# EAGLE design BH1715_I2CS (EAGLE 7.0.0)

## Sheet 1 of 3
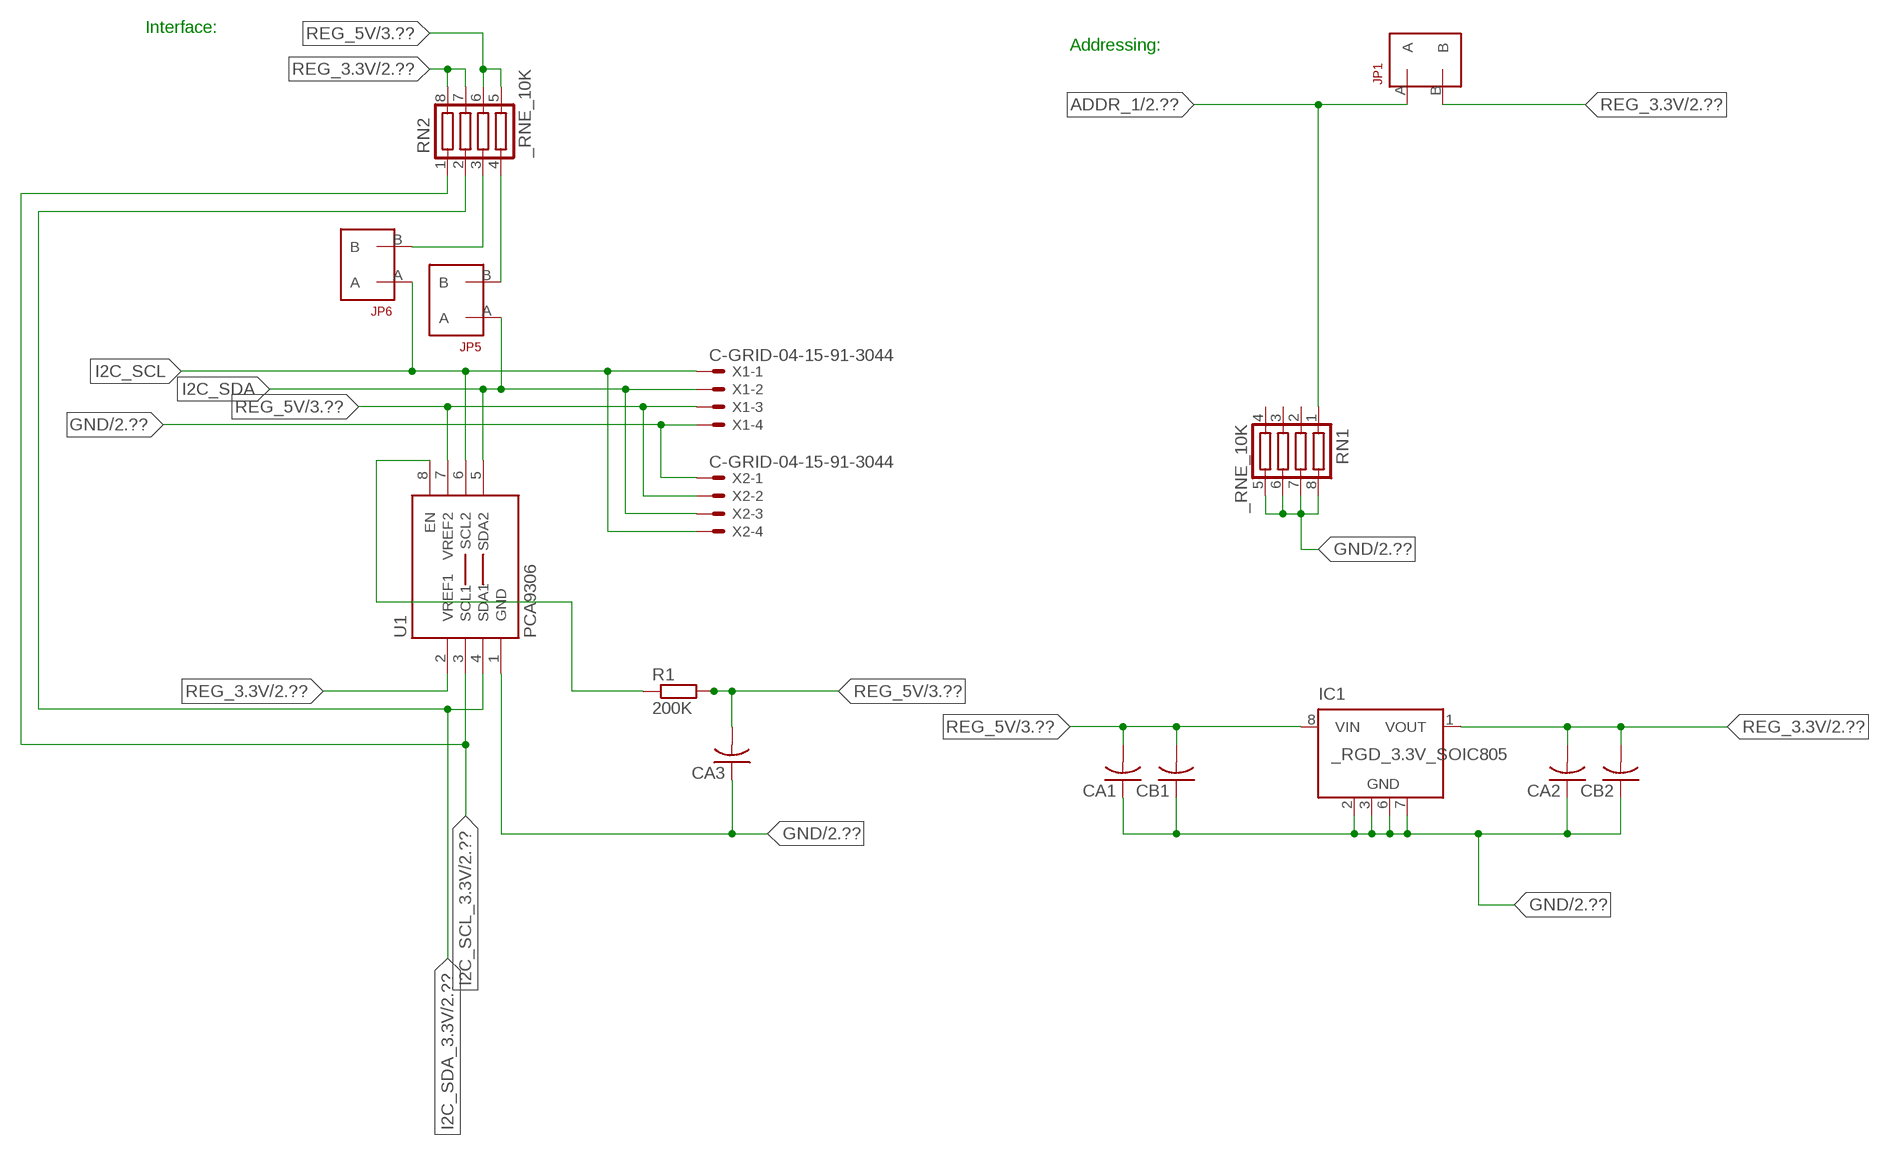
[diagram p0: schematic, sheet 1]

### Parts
CA1  CC1206KRX7R9BB104  [.1UF]
CA2  CC1206KRX7R9BB104  [.1UF]
CA3  CC1206KRX7R9BB104  [.1UF]
CB1  TMK316F106ZL-TC1206K  [TMK316F106ZL-T]
CB2  TMK316F106ZL-TC1206K  [TMK316F106ZL-T]
IC1  _RGD_3.3V_SOIC805  [_RGC_3.3V_SOIC8]
JP1  JUMPER_1X2_2MM  [JUMPER_1X2_2MM]
JP5  JUMPER_1X2_2MM  [JUMPER_1X2_2MM]
JP6  JUMPER_1X2_2MM  [JUMPER_1X2_2MM]
R1  200K  RESISTOR_SMT-0603  [R603]
RN1  _RNE_10K  [RNE]
RN2  _RNE_10K  [RNE]
U1  PCA9306  PCA9306_NCD  [PSOP-8]
X1  C-GRID-04-15-91-3044  [15-91-04]
X2  C-GRID-04-15-91-3044  [15-91-04]

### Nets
ADDR_1: JP1.A RN1.1 ; also sheet 2
GND: CA1.1 CA2.1 CA3.1 CB1.1 CB2.1 IC1.2(GND) IC1.3(GND) IC1.6(GND) IC1.7(GND) RN1.5 RN1.6 RN1.7 RN1.8 U1.1(GND) X1.4 X2.1 ; also sheet 2,3
I2C_SCL: JP6.A U1.6(SCL2) X1.1 X2.4
I2C_SCL_3.3V: RN2.1 U1.3(SCL1) ; also sheet 2
I2C_SDA: JP5.A U1.5(SDA2) X1.2 X2.3
I2C_SDA_3.3V: RN2.2 U1.4(SDA1) ; also sheet 2
N$1: JP6.B RN2.3
N$2: JP5.B RN2.4
N$23: R1.1 U1.8(EN)
REG_3.3V: CA2.2 CB2.2 IC1.1(VOUT) JP1.B RN2.7 RN2.8 U1.2(VREF1) ; also sheet 2
REG_5V: CA1.2 CA3.2 CB1.2 IC1.8(VIN) R1.2 RN2.5 RN2.6 U1.7(VREF2) X1.3 X2.2 ; also sheet 3
Unconnected: IC1.4(NC) IC1.5(NC) RN1.2 RN1.3 RN1.4

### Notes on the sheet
- Interface:
- Addressing:

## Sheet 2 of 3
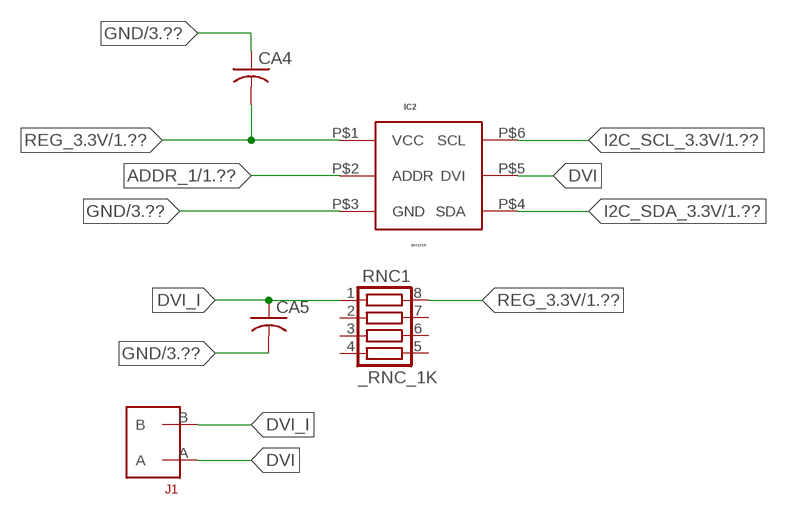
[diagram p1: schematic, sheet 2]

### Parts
CA4  _CA_.10UF_50VC1206K  [_CA_.1UF_50V]
CA5  _CA_.10UF_50VC1206K  [_CA_.1UF_50V]
IC2  BH1715  [BH1715]
J1  JUMPER_1X2_2MM  [JUMPER_1X2_2MM]
RNC1  _RNC_1K  [RNC]

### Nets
ADDR_1: IC2.P$2(ADDR) ; also sheet 1
DVI: IC2.P$5(DVI) J1.A
DVI_I: CA5.1 J1.B RNC1.1
GND: CA4.1 CA5.2 IC2.P$3(GND) ; also sheet 1,3
I2C_SCL_3.3V: IC2.P$6(SCL) ; also sheet 1
I2C_SDA_3.3V: IC2.P$4(SDA) ; also sheet 1
REG_3.3V: CA4.2 IC2.P$1(VCC) RNC1.8 ; also sheet 1
Unconnected: RNC1.2 RNC1.3 RNC1.4 RNC1.5 RNC1.6 RNC1.7

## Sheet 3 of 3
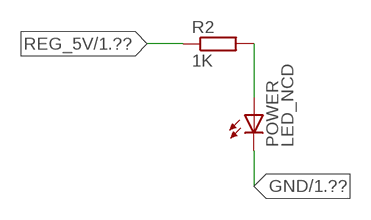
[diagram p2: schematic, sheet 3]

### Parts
POWER  LED_NCD  [CHIPLED_0603]
R2  1K  RESISTOR_SMT-0402  [R402]

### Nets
GND: POWER.C ; also sheet 1,2
N$4: POWER.A R2.2
REG_5V: R2.1 ; also sheet 1

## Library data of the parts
CA1-CA3 = NCD_ULTIMATE_LIBRARY:CC1206KRX7R9BB104: Capacitor CA .1uF 50V SMT C1206K CC1206KRX7R9BB104
CA4 CA5 = NCD_ULTIMATE_LIBRARY:_CA_.10UF_50V: Capacitor .1uF SMT
CB1 CB2 = NCD_ULTIMATE_LIBRARY:TMK316F106ZL-T: Capacitor CB 10uF SMT 1206 TMK316F106ZL-T
IC1 = NCD_ULTIMATE_LIBRARY:_RGD_3.3V_SOIC8: Regulator Linear 3.3V Chip Positive VOLTAGE REGULATOR Digikey 497-1199-2-ND/L78L33ACD13TR
IC2 = NCD_ULTIMATE_bhaskar:BH1715: Digikey BH1715FVCDKR-ND/BH1715FVC-TR
J1 JP1 JP5 JP6 = NCD_ULTIMATE_CONNECTORS:JUMPER_1X2_2MM
POWER = NCD_ULTIMATE_LIBRARY:LED_NCD: LED Digikey 754-1132-2-ND/APT2012SRCPRV
R1 R2 = NCD_ULTIMATE_LIBRARY:RESISTOR_SMT: NCD Resistor
RN1 RN2 = NCD_ULTIMATE_LIBRARY:_RNE_10K: Resistor Array RNE SMT 10K x 4 Single Resistor Source: http://www.ctscorp.com/components/Datasheets/CTSChipArrayDs.pdf Digikey 742C083103JPTR-ND/742C083103JP; OC_FARNELL: unknown; OC_NEWARK: unknown
RNC1 = NCD_ULTIMATE_LIBRARY:_RNC_1K: Resistor Array RNC SMT 1K x 4 Single Resistor Source: http://www.ctscorp.com/components/Datasheets/CTSChipArrayDs.pdf Digikey 742C083102JPTR-ND/742C083102JP; OC_FARNELL: unknown; OC_NEWARK: unknown
U1 = NCD_ULTIMATE_LIBRARY:PCA9306_NCD: NCD Bidirectional I2C level shifter. NOT compatible with all available part number pinout schemes- DOUBLE CHECK!!!; PROD_ID: IC-10023
X1 X2 = NCD_ULTIMATE_CONNECTORS:C-GRID-04: CONNECTOR 4-Pos I2C wire to board 2.54 mm (0.100") pitch header Digikey WM1342-ND/0015912045; OC_FARNELL: unknown; OC_NEWARK: unknown

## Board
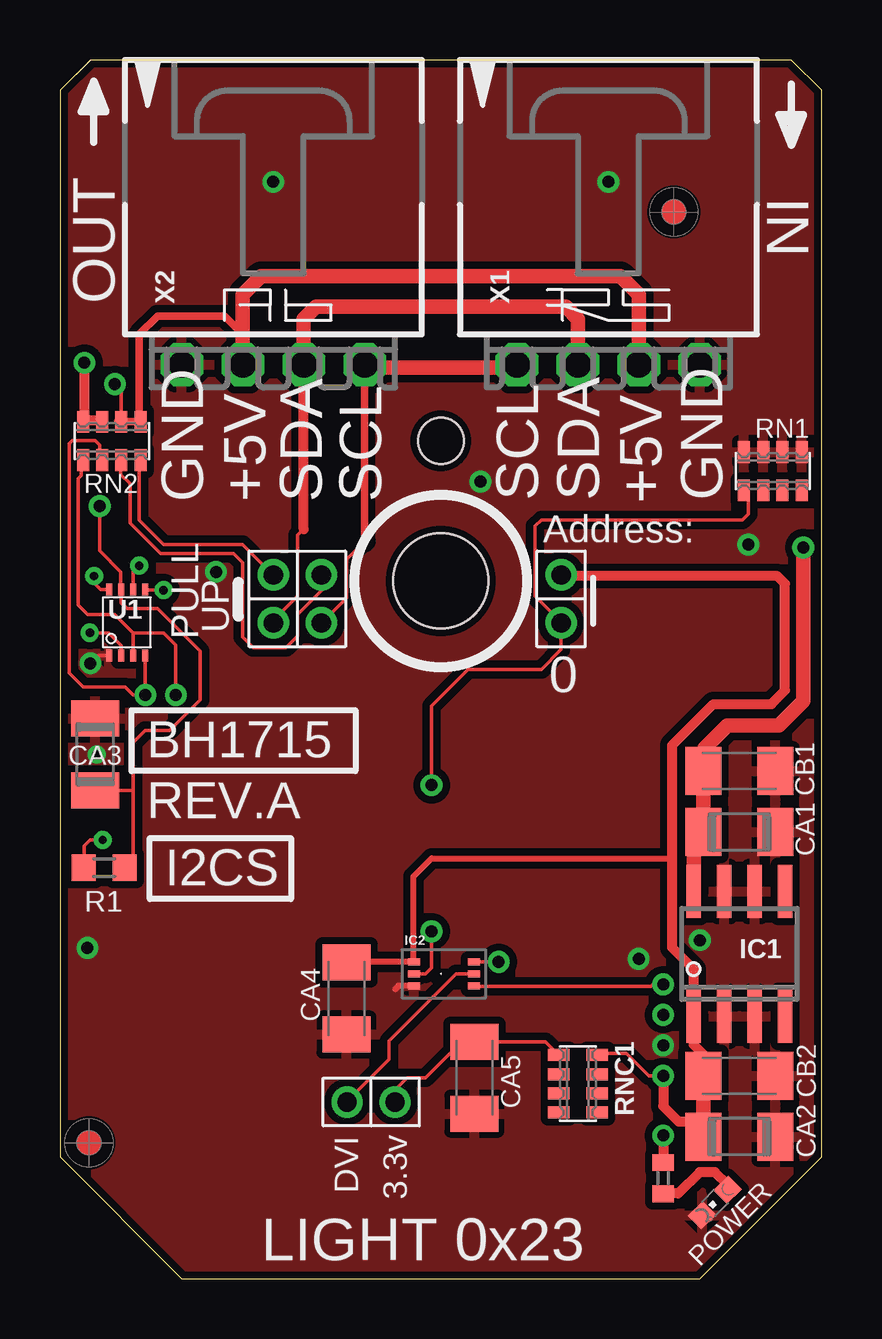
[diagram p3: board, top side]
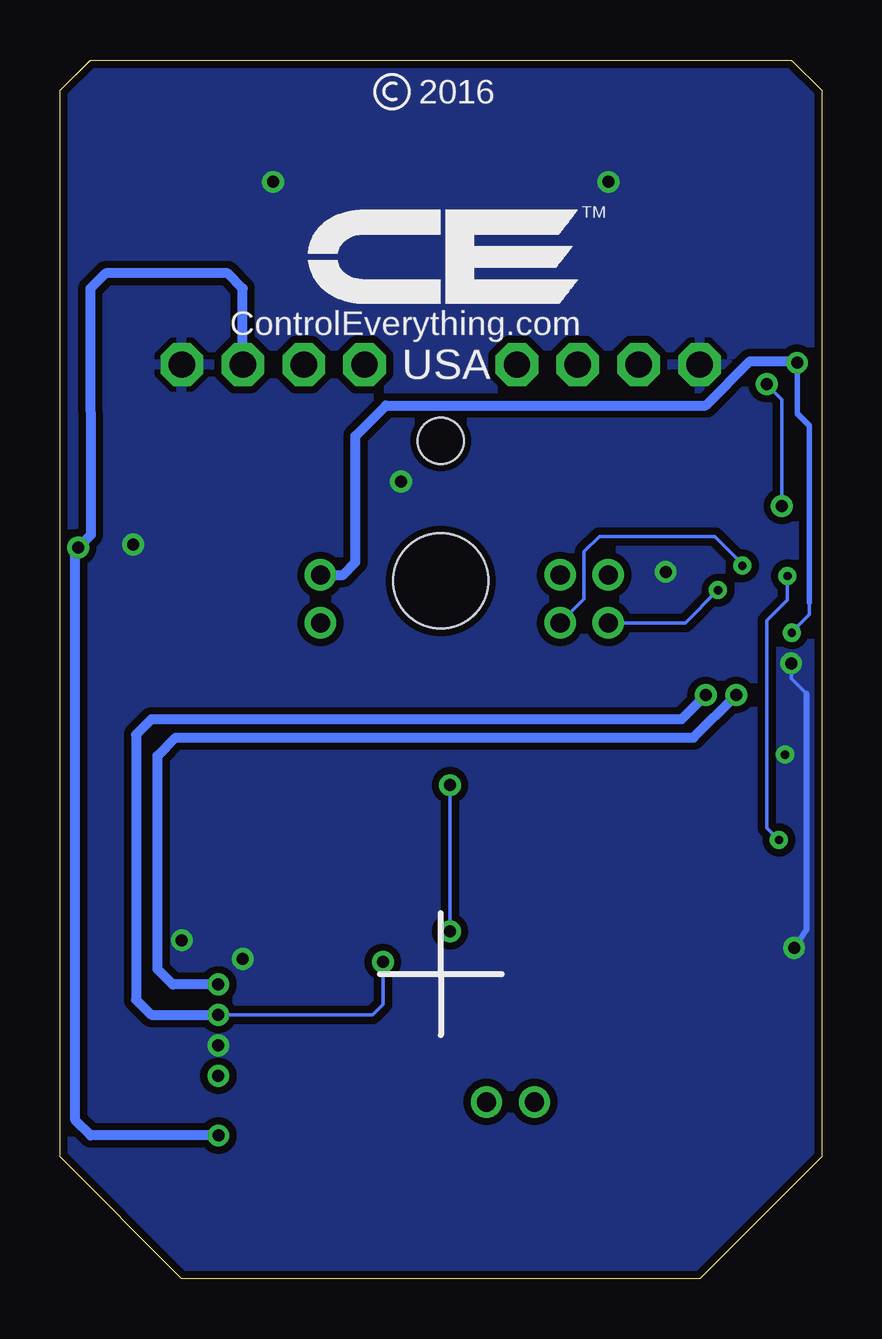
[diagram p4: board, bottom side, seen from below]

Size 31.75 x 50.8 mm. Coordinates in mm from the lower left corner, seen from the top.
Outline: 32 segments
Copper layers (1*16): Top 0.035mm / dielectric 1.5mm / Bottom 0.035mm
Design rules "default": minimum track width 5mil, minimum drill 24mil, track to track 5mil, track to pad 5mil, pad to pad 5mil, via to via 5mil, smd to smd 5mil, copper to edge 10mil, drill to drill 8mil, minimum pad ring 10mil, minimum via ring 8mil, stop-mask expansion 2mil, vias tented up to drill 0mil, thermal gap 10mil
Holes 3.96 mm at 15.88,29.08
Holes 1.91 mm at 15.88,34.93

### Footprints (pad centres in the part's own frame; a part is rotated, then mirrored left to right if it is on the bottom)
.1UF = smd 1.5 x 2: 1 -1.5,0; 2 1.5,0
_CA_.1UF_50V = smd 1.5 x 2: 1 -1.5,0; 2 1.5,0
TMK316F106ZL-T = smd 1.5 x 2: 1 -1.5,0; 2 1.5,0
_RGC_3.3V_SOIC8 = smd 0.6 x 2.2: 1 -1.905,-2.6; 2 -0.635,-2.6; 3 0.635,-2.6; 4 1.905,-2.6; 5 1.905,2.6; 6 0.635,2.6; 7 -0.635,2.6; 8 -1.905,2.6
BH1715 = smd 0.5 x 0.3: P$1 -1.5,0; P$2 -1.5,-0.5; P$3 -1.5,-1; P$4 1,-1; P$5 1,-0.5; P$6 1,0
JUMPER_1X2_2MM = drill 0.8: A 0,2; B 0,0
CHIPLED_0603 = smd 0.8 x 0.876: A 0,-0.75; C 0,0.75
R603 = smd 1 x 1.1: 1 -0.85,0; 2 0.85,0
R402 = smd 0.7 x 0.9: 1 -0.65,0; 2 0.65,0
RNE = smd 0.5 x 0.9: 1 -1.2,-0.8; 2 -0.4,-0.8; 3 0.4,-0.8; 4 1.2,-0.8; 5 1.2,0.8; 6 0.4,0.8; 7 -0.4,0.8; 8 -1.2,0.8
RNC = smd 0.5 x 0.9: 1 -1.2,-0.8; 2 -0.4,-0.8; 3 0.4,-0.8; 4 1.2,-0.8; 5 1.2,0.8; 6 0.4,0.8; 7 -0.4,0.8; 8 -1.2,0.8
PSOP-8 = smd 0.25 x 0.5: 1 -0.73,-1.37; 2 -0.23,-1.37; 3 0.27,-1.37; 4 0.77,-1.37; 5 0.77,1.38; 6 0.27,1.38; 7 -0.23,1.38; 8 -0.73,1.38
15-91-04 = drill 1.1 pad 1.778 octagon: 1 -3.81,-7.62; 2 -1.27,-7.62; 3 1.27,-7.62; 4 3.81,-7.62

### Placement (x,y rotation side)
CA1  28.32,18.62 180 top
CA2  28.32,5.92 180 top
CA3  1.46,21.86 270 top
CA4  11.94,11.68 90 top
CA5  17.27,8.38 270 top
CB1  28.32,21.16 180 top
CB2  28.32,8.46 180 top
IC1  28.32,13.54 0 top
IC2  16.26,13.21 0 top
J1  13.97,7.37 90 top
JP1  20.89,29.34 180 top
JP5  8.89,29.34 180 top
JP6  10.9,29.34 180 top
POWER  27.3,3.18 135 top
R1  1.84,17.13 0 top
R2  25.15,4.19 270 top
RN1  29.72,33.66 0 top
RN2  2.16,34.93 0 top
RNC1  21.59,8.13 270 top
U1  2.79,27.36 0 top
U$5  [VISION_REF10]  1.21,5.66 90 top
U$28  [VISION_REF10]  25.59,44.46 90 top
X1  22.86,45.72 0 top
X2  8.89,45.72 0 top

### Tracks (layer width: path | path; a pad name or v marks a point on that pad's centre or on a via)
ADDR_1  (via drill 0.5)
  Top 0.152: RN1.1 28.7,32.78 28.7,31.88 28.45,31.62 20.07,31.62 19.81,31.37 19.81,28.45 20.89,27.37 JP1.A 20.89,26.23 20.07,25.4 17.02,25.4 15.49,23.88 v15.49,20.57 | IC2.P$2 15.24,12.7 15.49,12.95 v15.49,14.48
  Bottom 0.152: v15.49,14.48 v15.49,20.57
DVI
  Top 0.152: IC2.P$5 17.25,12.7 16.51,12.7 13.72,9.91 13.72,9.14 11.97,7.4 J1.A
DVI_I
  Top 0.152: J1.B 13.97,7.87 14.48,8.38 15.24,8.38 16.26,9.4 16.79,9.4 CA5.1 20.24,9.88 RNC1.1
GND  (via drill 0.35, 0.5)
  Top 0.152: CA3.1 1.52,23.42 1.52,23.62 | v1.27,25.65 1.6,25.99 U1.1
  Top 0.254: IC2.P$3 14.11,12.21 13.97,12.07
  Bottom 0.152: 0.64,24.38 1.27,25.02 v1.27,25.65
  Bottom 0.254: 0.64,24.38 0.64,14.56 v1.15,13.79
  other vias: 8.89,45.72 22.86,45.72 25.15,9.73 17.53,33.22 26.67,14.11 6.5,29.46 24.13,13.34 1.52,21.84 28.7,30.61
  pour Bottom (isolate 0.305): -0.64,5.08 -0.64,49.53 1.27,51.44 30.48,51.44 32.38,49.53 32.38,5.08 26.67,-0.63 5.08,-0.63
  pour Top (isolate 0.305): 4.45,-1.27 -1.27,4.45 -1.27,50.17 0.64,52.07 31.11,52.07 33.02,50.17 33.02,4.45 27.3,-1.27
I2C_SCL  (via drill 0.35)
  Top 0.152: 12.7,30.73 11.94,29.97 11.94,28.38 JP6.A | v3.3,29.72 3.06,29.48 U1.6
  Top 0.305: 12.7,30.73 X2.4
  Top 0.406: X2.4 12.7,37.97 | 19.05,37.97 X1.1
  Top 0.61: 12.7,37.97 19.05,37.97
  Bottom 0.152: JP6.A 9.91,28.33 9.91,30.3 9.27,30.94 4.45,30.94 3.3,29.79 v3.3,29.72
I2C_SCL_3.3V  (via drill 0.5)
  Top 0.152: RN2.1 0.89,34.07 0.89,33.48 0.77,33.35 0.77,28.08 1.16,27.69 2.29,27.69 3.06,26.91 | IC2.P$6 v18.29,13.21 | 3.06,26.91 U1.3 | v4.83,24.33 v4.83,24.34 4.83,26.42 4.33,26.91 3.06,26.91
  Bottom 0.152: v18.29,13.21 18.29,11.43 18.72,11 v25.15,11
  Bottom 0.406: v4.83,24.33 5.84,23.32 27.94,23.32 28.58,22.68 28.58,11.63 27.94,11 v25.15,11
I2C_SDA  (via drill 0.35)
  Top 0.152: JP5.A 8.89,27.44 9.91,28.45 9.91,30.99 10.16,31.24 | U1.5 3.6,28.7 v4.32,28.7
  Top 0.406: 10.16,31.24 10.16,31.25 10.16,38.74
  Top 0.61: X2.3 10.16,38.74 10.16,40.01 10.67,40.51 21.09,40.51 21.59,40.01 X1.2
  Bottom 0.152: v4.32,28.7 5.68,27.34 JP5.A
I2C_SDA_3.3V  (via drill 0.5)
  Top 0.152: RN2.2 1.65,34.14 1.65,34.75 1.46,34.94 0.51,34.94 0.38,34.81 0.38,26.37 0.38,26.36 0.38,25.25 0.96,24.66 2.72,24.66 3.05,24.33 v3.56,24.33 v3.56,24.34 U1.4 | IC2.P$4 17.27,12.19 24.64,12.19 24.71,12.27 v25.15,12.27
  Bottom 0.406: v25.15,12.27 27.05,12.27 27.69,12.9 27.69,21.79 26.93,22.56 5.34,22.56 v3.56,24.33
N$1
  Top 0.152: JP6.B 10.92,29.31 10.92,28.7 9.91,27.69 9.91,26.8 9.42,26.31 8.06,26.31 7.62,26.75 7.62,29.84 7.24,30.23 4.19,30.23 2.92,31.5 2.92,33.15 2.54,33.53 2.54,34.1 RN2.3
  Top 0.305: 2.54,34.02 RN2.3
N$2
  Top 0.152: JP5.B 7.62,30.61 4.32,30.61 3.3,31.62 3.3,34.07 RN2.4
  Top 0.305: 3.37,33.88 RN2.4
N$4
  Top 0.406: POWER.A 27.84,3.92 27.3,4.45 26.67,4.45 25.78,3.56 25.16,3.56 R2.2
N$23  (via drill 0.35)
  Top 0.152: R1.1 1.02,17.16 1.02,18.03 1.27,18.29 v1.78,18.29 | U1.8 1.69,28.74 1.42,29.01 v1.42,29.29
  Bottom 0.152: v1.78,18.29 2.29,18.8 2.29,27.43 1.42,28.3 v1.42,29.29
REG_3.3V  (via drill 0.35, 0.5)
  Top 0.152: 12.45,13.21 12.42,13.18 CA4.2 | IC2.P$1 14.73,13.23 | RNC1.8 22.46,9.4 23.62,9.4 24.56,8.46 v25.15,8.46 | v1.25,26.92 2.03,26.92 2.56,26.4 U1.2
  Top 0.254: IC2.P$1 12.45,13.21 | 25.53,17.53 15.49,17.53 14.73,16.76 14.73,13.23 | JP1.B 20.95,29.34 21,29.29
  Top 0.406: CB2.2 26.82,9.35 26.42,9.75 26.42,10.36 | v25.15,8.46 25.15,7.19 25.78,6.55 26.82,6.55 | IC1.1 26.42,12.9 25.53,13.79 25.53,17.53 25.53,22.24 27.24,23.95 29.66,23.95 30.23,24.52 30.23,28.97 29.91,29.29 21,29.29 | 26.52,5.62 CA2.2 | v1.02,38.18 1.02,35.78 | 1.02,35.78 RN2.8 | 1.02,35.78 1.71,35.78 RN2.7
  Top 0.61: CB2.2 26.82,6.55 CA2.2 | 26.42,10.36 IC1.1
  Bottom 0.152: 0.51,28.19 0.51,27.69 1.14,27.05 v1.25,26.92
  Bottom 0.229: 0.51,28.19 0.51,35.56 1.02,36.07 v1.02,38.18
  Bottom 0.406: v1.02,38.18 1.08,38.24 2.99,38.24 4.83,36.4 18.16,36.4 19.43,35.13 19.43,29.87 19.94,29.34 JP1.B
REG_5V  (via drill 0.5)
  Top 0.152: RN2.6 2.56,37.01 v2.29,37.29 | R1.2 3.05,17.49 3.05,20.36 | 3.05,20.36 3.05,22.35 3.56,22.86 4.57,22.86 5.84,24.13 5.84,26.16 4.06,27.94 2.79,27.94 2.56,28.17 U1.7 2.54,28.76 2.54,29.46 1.65,30.35 v1.65,32.21 | CA3.2 3.05,20.36
  Top 0.305: 7.62,39.37 7.5,39.37 | 2.42,35.74 RN2.6 RN2.5 3.31,35.8 3.31,39.37 4.07,40.13 6.86,40.13 7.62,39.37 | X2.2 7.62,39.37
  Top 0.406: v25.15,5.97 R2.1
  Top 0.61: X2.2 7.62,41.02 8.38,41.78 23.37,41.78 24.13,41.02 X1.3 | IC1.8 26.42,18.21 CA1.2 CB1.2 26.86,21.2 26.86,22.11 27.82,23.06 29.98,23.06 30.99,24.08 v30.99,30.48
  Bottom 0.152: v1.65,32.21 1.65,36.65 v2.29,37.29
  Bottom 0.406: X1.3 24.13,41.28 24.77,41.91 29.84,41.91 30.48,41.27 30.47,31 v30.99,30.48 31.11,30.36 31.11,6.6 30.48,5.97 v25.15,5.97

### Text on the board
tPlace: LIGHT 0x23
tNames: IN | OUT | GND | +5V | SDA | SCL | SCL | SDA | +5V | GND | Address: | PULL | UP | 0 | BH1715 | REV.A | I2CS | DVI | 3.3v
bNames: 2016 | TM | ControlEverything.com | USA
